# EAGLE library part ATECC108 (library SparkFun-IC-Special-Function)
ATECC108 ECDSA with NIST ATECC108: Provides ECDSA with NIST curves P256, B283, and K283. Also, a RNG, 8.5Kb EEPROM. 2.0V - 5.5V. Datasheet SparkFun Products CryptoCape (DEV-12773) SparkFun CryptoShield (DEV-13183)
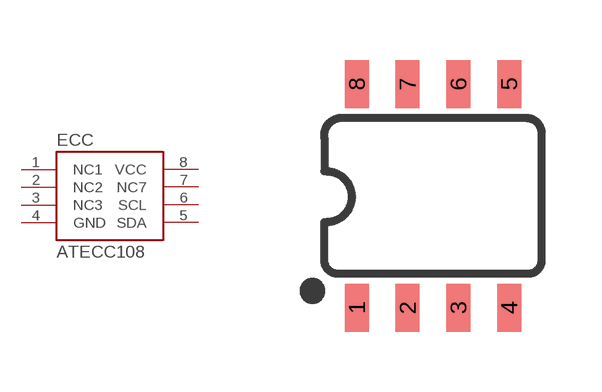
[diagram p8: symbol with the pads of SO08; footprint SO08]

Designator prefix ECC

## ATECC108 (PROD_ID: IC-11982; VALUE: ATECC108)  [SO08]
1  NC1
2  NC2  nc
3  NC3  nc
4  GND  pwr
5  SDA
6  SCL
7  NC7  nc
8  VCC  pwr

## Footprint SO08 (pad centres in mm)
SOIC, 0.15 inch width
smd 0.6 x 1.2: 1 -1.905,-2.8; 2 -0.635,-2.8; 3 0.635,-2.8; 4 1.905,-2.8; 5 1.905,2.8; 6 0.635,2.8; 7 -0.635,2.8; 8 -1.905,2.8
